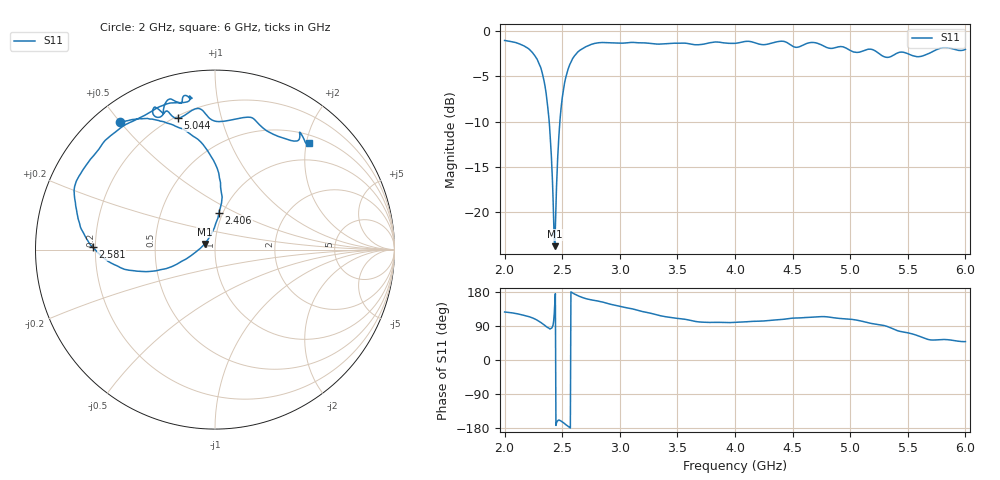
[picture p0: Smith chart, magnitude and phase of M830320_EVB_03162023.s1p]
# Hz S RI R 50
! CMT, M5090, 19127454, 21.2.4/2
! Date: 3/16/2023 5:10:47 PM
! Data: Format (Calibration Info)
! Freq	S11:Re/Im(F2 Pxt)
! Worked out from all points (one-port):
!   800 points, 2 GHz to 6 GHz, reference 50 ohm
!   lowest |S11| = -23.7 dB at 2.436 GHz (marker M1), VSWR 1.14, Z = 44.6 + j2.87 ohm
!   |S11| at or under -10 dB: 2.387 GHz to 2.48 GHz (92.74 MHz wide, 3.81 % of centre)
!   S11 on the Smith chart (normalised r, x): 2 GHz: 0.08, +0.50; 2.406 GHz: 0.96, +0.41; 2.581 GHz: 0.19, +0.01; 5.044 GHz: 0.21, +0.73; 6 GHz: 0.65, +2.05
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2e9  -0.5287 0.709
2.185232e9  -0.3634 0.7274
2.300375e9  -0.1352 0.6419
2.365457e9  0.0211 0.425
2.405507e9  0.0219 0.2052
2.420526e9  -0.00418 0.1195
2.435544e9  -0.0567 0.032
2.450563e9  -0.1334 -0.0337
2.475594e9  -0.2723 -0.106
2.500626e9  -0.4106 -0.1214
2.580726e9  -0.6822 0.0132
2.645807e9  -0.7578 0.1553
2.77597e9  -0.7853 0.3258
3.001252e9  -0.6702 0.5304
3.206508e9  -0.5184 0.6836
3.501877e9  -0.29 0.8034
3.702128e9  -0.1473 0.8268
4.002503e9  -0.1389 0.8415
4.403004e9  -0.2531 0.8385
4.503129e9  -0.2878 0.7682
4.748436e9  -0.347 0.7619
5.003755e9  -0.2346 0.7405
5.043805e9  -0.2087 0.7315
5.178974e9  -0.0924 0.7862
5.50438e9  0.2371 0.707
5.704631e9  0.4605 0.6065
5.819775e9  0.4732 0.6536
6e9  0.5223 0.5914
